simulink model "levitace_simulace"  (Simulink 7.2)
settings: Solver=ode45  StartTime=0.0  StopTime=10  RelTol=1e-3
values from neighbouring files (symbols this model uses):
  g = 9.81    [podklad.m]    (also in kockaLQG.m; kockaLQR.m; nadrze_soustava.m; nadoby.m)
  kc = kf/(ki^2)    (= 5.56473829201e-06)    [podklad.m]
  Kfv = 0.02    [podklad.m]
  ki = 0.33    [podklad.m]
  Kreg3 = lqg(sys,0.0001*eye(4),QMV,10000)    [podklad.m]
  mk = 8.37e-3    (= 0.00837)    [podklad.m]    (also in kockaLQG.m = 1; kockaLQR.m = 1)
  Ta = 3e-3    (= 0.003)    [podklad.m]
  x0 = 8.26e-3    (= 0.00826)    [podklad.m]
undefined symbols (not defined in the file or in its folder): float
libraries: simulink x2

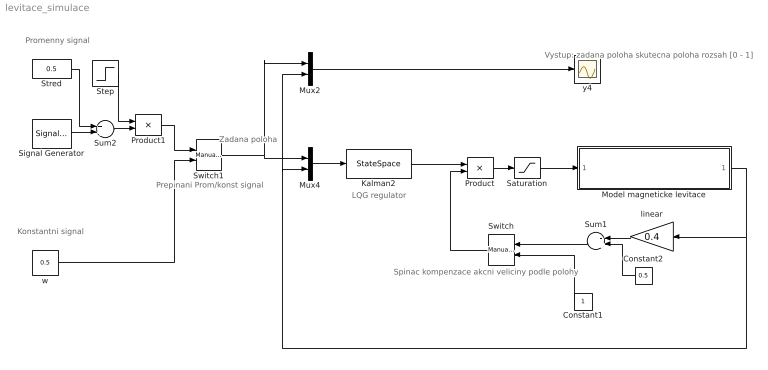
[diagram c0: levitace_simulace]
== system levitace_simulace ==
  note: Promenny signal
  note: Konstantni signal
  note: Prepinani Prom/konst signal
  note: Spinac kompenzace akcni veliciny podle polohy
  note: LQG regulator
  note: Zadana poloha
  note: Vystup: zadana poloha skutecna poloha rozsah [0 - 1]
  Constant1 : Constant  Orientation=left  OutDataType=sfix(16)  OutScaling=2^0
  Constant2 : Constant  Orientation=left  Value=0.5  OutDataType=sfix(16)  OutScaling=2^0
  Kalman2 : StateSpace  A=Kreg3.a  B=Kreg3.b  C=Kreg3.c  D=Kreg3.d
  Model magneticke levitace : Subsystem
  Mux2 : Mux  Inputs=2
  Mux4 : Mux  Inputs=2
  Product : Product  OutDataType=sfix(16)  OutScaling=2^0
  Product1 : Product  OutDataType=sfix(16)  OutScaling=2^0
  Saturation : Saturate  UpperLimit=1  LowerLimit=0
  Signal Generator : SignalGenerator  WaveForm=square  Amplitude=0.200  Frequency=0.5
  Step : Step  Time=0  SampleTime=0
  Stred : Constant  Value=0.5  OutDataType=sfix(16)  OutScaling=2^0
  Sum1 : Sum  Orientation=left  Inputs=-+  OutDataType=sfix(16)  OutScaling=2^0
  Sum2 : Sum  OutDataType=sfix(16)  OutScaling=2^0
  Switch : simulink/Signal Routing/Manual Switch  Orientation=left  SystemSampleTime=-1  sw=0  action=0  varsize=off
  Switch1 : simulink/Signal Routing/Manual Switch  SystemSampleTime=-1  sw=1  action=0  varsize=off
  linear : Gain  Orientation=left  Gain=0.4  ParameterDataType=sfix(16)  ParameterScaling=2^0  OutDataType=sfix(16)  OutScaling=2^0
  w : Constant  Value=0.5  OutDataType=sfix(16)  OutScaling=2^0
  y4 : Scope
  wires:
  Kalman2/1 -> Product/1
  Product/1 -> Saturation/1
  linear/1 -> Sum1/1
  Constant2/1 -> Sum1/2
  Sum1/1 -> Switch/1
  Switch/1 -> Product/2
  Stred/1 -> Sum2/1
  Signal Generator/1 -> Sum2/2
  w/1 -> Switch1/2
  Model magneticke levitace/1(y - vystupni napeti) -> linear/1, Mux4/2, Mux2/2
  Product1/1 -> Switch1/1
  Sum2/1 -> Product1/2
  Step/1 -> Product1/1
  Switch1/1 -> Mux4/1, Mux2/1
  Mux4/1 -> Kalman2/1
  Constant1/1 -> Switch/2
  Mux2/1 -> y4/1
  Saturation/1 -> Model magneticke levitace/1(u -vstupni napeti)

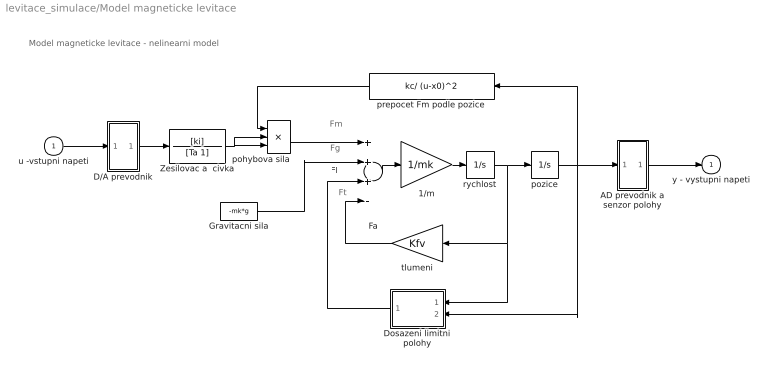
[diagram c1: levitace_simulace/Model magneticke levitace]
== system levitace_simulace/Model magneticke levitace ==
  note: Model magneticke levitace - nelinearni model
  note: Fm
  note: Fg
  note: Ft
  note: Fl
  u -vstupni napeti : Inport  OutDataType=sfix(16)  OutScaling=2^0
  1/m : Gain  Gain=1/mk  ParameterDataType=sfix(16)  ParameterScaling=2^0  OutDataType=sfix(16)  OutScaling=2^0
  AD prevodnik a senzor polohy : Subsystem
  D/A prevodnik : Subsystem
  Dosazeni limitni polohy : Subsystem  Orientation=left
  Fa : Sum  Inputs=+++-  OutDataType=sfix(16)  OutScaling=2^0
  Gravitacni sila : Constant  Value=-mk*g  OutDataType=sfix(16)  OutScaling=2^0
  Zesilovac a  civka : TransferFcn  Numerator=[ki]  Denominator=[Ta 1]
  pohybova sila : Product  Inputs=3  OutDataType=sfix(16)  OutScaling=2^0
  pozice : Integrator  LimitOutput=on  UpperSaturationLimit=0.005  LowerSaturationLimit=0
  prepocet Fm podle pozice : Fcn  Orientation=left  Expr=kc/ (u-x0)^2
  rychlost : Integrator
  tlumeni : Gain  Orientation=left  Gain=Kfv  ParameterDataType=sfix(16)  ParameterScaling=2^0  OutDataType=sfix(16)  OutScaling=2^0
  y - vystupni napeti : Outport
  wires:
  Zesilovac a  civka/1 -> pohybova sila/2, pohybova sila/3
  Dosazeni limitni polohy/1(force) -> Fa/3
  pozice/1 -> AD prevodnik a senzor polohy/1(in_1), prepocet Fm podle pozice/1, Dosazeni limitni polohy/2(position)
  AD prevodnik a senzor polohy/1(out_1) -> y - vystupni napeti/1
  u -vstupni napeti/1 -> D/A prevodnik/1(in_1)
  D/A prevodnik/1(out_1) -> Zesilovac a  civka/1
  Gravitacni sila/1 -> Fa/2
  pohybova sila/1 -> Fa/1
  Fa/1 -> 1/m/1
  1/m/1 -> rychlost/1
  prepocet Fm podle pozice/1 -> pohybova sila/1
  tlumeni/1 -> Fa/4
  rychlost/1 -> pozice/1, Dosazeni limitni polohy/1(velocity), tlumeni/1

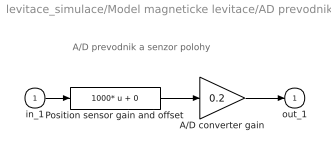
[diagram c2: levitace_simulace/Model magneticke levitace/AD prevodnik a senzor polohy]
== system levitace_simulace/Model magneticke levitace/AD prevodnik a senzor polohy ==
  note: A/D prevodnik a senzor polohy
  in_1 : Inport  OutDataType=sfix(16)  OutScaling=2^0
  A/D converter gain : Gain  Gain=0.2  ParameterDataType=sfix(16)  ParameterScaling=2^0  OutDataType=sfix(16)  OutScaling=2^0
  Position sensor gain and offset : Fcn  Expr=1000* u + 0
  out_1 : Outport
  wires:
  A/D converter gain/1 -> out_1/1
  Position sensor gain and offset/1 -> A/D converter gain/1
  in_1/1 -> Position sensor gain and offset/1

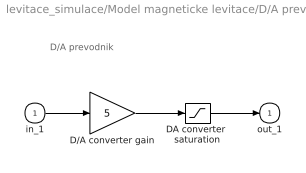
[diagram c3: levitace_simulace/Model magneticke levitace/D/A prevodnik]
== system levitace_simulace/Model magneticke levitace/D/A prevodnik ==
  note: D/A prevodnik
  in_1 : Inport  OutDataType=sfix(16)  OutScaling=2^0
  D/A converter gain : Gain  Gain=5  ParameterDataType=sfix(16)  ParameterScaling=2^0  OutDataType=sfix(16)  OutScaling=2^0
  DA converter  saturation : Saturate  UpperLimit=5  LowerLimit=-5
  out_1 : Outport
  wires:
  D/A converter gain/1 -> DA converter  saturation/1
  DA converter  saturation/1 -> out_1/1
  in_1/1 -> D/A converter gain/1

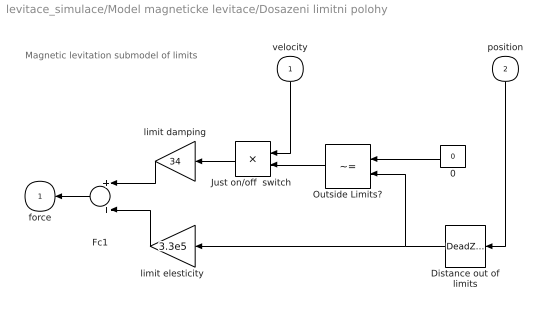
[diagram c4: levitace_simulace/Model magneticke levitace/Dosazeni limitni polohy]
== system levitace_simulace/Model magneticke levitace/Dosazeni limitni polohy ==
  note: Magnetic levitation submodel of limits
  velocity : Inport  Orientation=down  OutDataType=sfix(16)  OutScaling=2^0
  position : Inport  Orientation=down  Port=2  OutDataType=sfix(16)  OutScaling=2^0
  0 : Constant  Orientation=left  Value=0  OutDataType=sfix(16)  OutScaling=2^0
  Distance out of limits : DeadZone  Orientation=left  LowerValue=0  UpperValue=0.005
  Fc1 : Sum  Orientation=left  OutDataType=sfix(16)  OutScaling=2^0
  "Just on/off  switch " : Product  Orientation=left  OutDataType=sfix(16)  OutScaling=2^0
  Outside Limits? : RelationalOperator  Orientation=left  Operator=~=  LogicOutDataTypeMode=Specify via dialog  LogicDataType=float('double')  OutDataTypeStr=float('double')
  limit damping : Gain  Orientation=left  Gain=34  ParameterDataType=sfix(16)  ParameterScaling=2^0  OutDataType=sfix(16)  OutScaling=2^0
  limit elesticity : Gain  Orientation=left  Gain=3.3e5  ParameterDataType=sfix(16)  ParameterScaling=2^0  OutDataType=sfix(16)  OutScaling=2^0
  force : Outport  Orientation=left
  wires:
  position/1 -> Distance out of limits/1
  Fc1/1 -> force/1
  velocity/1 -> "Just on/off  switch "/1
  "Just on/off  switch "/1 -> limit damping/1
  0/1 -> Outside Limits?/1
  Outside Limits?/1 -> "Just on/off  switch "/2
  limit elesticity/1 -> Fc1/2
  limit damping/1 -> Fc1/1
  Distance out of limits/1 -> limit elesticity/1, Outside Limits?/2
